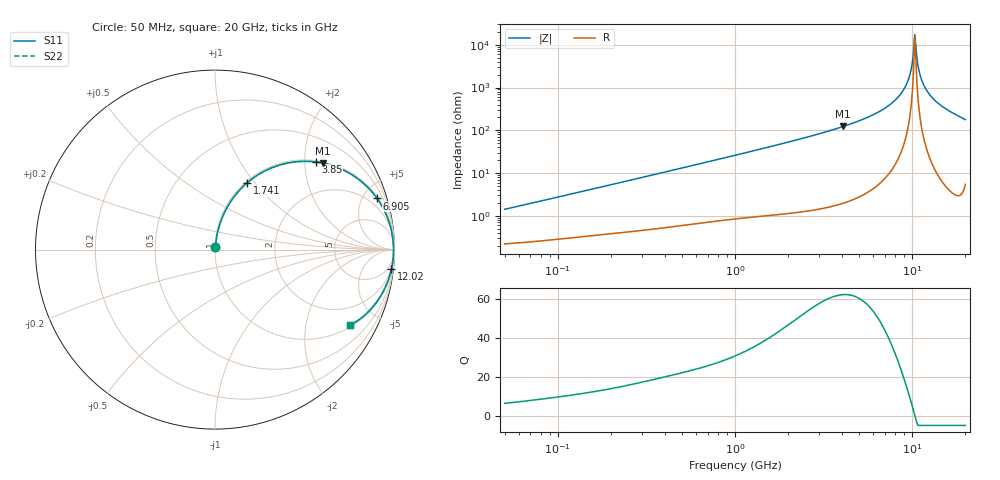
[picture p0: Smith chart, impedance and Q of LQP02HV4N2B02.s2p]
!Murata Part Number: LQP02HV4N2B02
!These Parameters are Measured in Series Mode Connection
!  o--[Z]--o
!Port1  Port2
!  o-------o
!Freq. Start=50[MHz] Stop=20[GHz], 401[Steps]
# Hz S RI R 50
!Freq.(Hz) S11(Real) S11(Imag) S21(Real) S21(Imag) S12(Real) S12(Imag) S22(Real) S22(Imag)
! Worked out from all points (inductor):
!   401 points, 50 MHz to 20 GHz, reference 50 ohm
!   read as one part in series: L = 4.42 nH near 51.52 MHz
!   highest Q = 62.3 at 4.088 GHz (marker M1), where L = 4.79 nH
!   self-resonance near 10.35 GHz
!   S11 on the Smith chart (normalised r, x): 50 MHz: 1.00, +0.03; 1.741 GHz: 1.02, +0.91; 3.85 GHz: 1.04, +2.27; 6.905 GHz: 1.14, +6.29; 12.02 GHz: 2, -18; 20 GHz: 1.11, -3.53
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5e7  0.0024 0.014  0.9976 -0.014  0.9976 -0.014  0.0024 0.014
1.364002e8  0.00457 0.0366  0.9954 -0.0366  0.9954 -0.0366  0.00457 0.0366
3.721004e8  0.0144 0.0959  0.9856 -0.0959  0.9856 -0.0959  0.0144 0.0959
1e9  0.07 0.2394  0.93 -0.2394  0.93 -0.2394  0.07 0.2394
1.740566e9  0.1787 0.3716  0.8213 -0.3716  0.8213 -0.3716  0.1787 0.3716
2.728004e9  0.3599 0.4711  0.6401 -0.4711  0.6401 -0.4711  0.3599 0.4711
3.850025e9  0.5619 0.4882  0.4381 -0.4882  0.4381 -0.4882  0.5619 0.4882
4.087748e9  0.6004 0.4819  0.3996 -0.4819  0.3996 -0.4819  0.6004 0.4819
5.515528e9  0.788 0.4001  0.212 -0.4001  0.212 -0.4001  0.788 0.4001
6.905011e9  0.903 0.2852  0.097 -0.2852  0.097 -0.2852  0.903 0.2852
7.442007e9  0.9325 0.2384  0.0675 -0.2384  0.0675 -0.2384  0.9325 0.2384
8.389408e9  0.9687 0.1569  0.0313 -0.1569  0.0313 -0.1569  0.9687 0.1569
9.178299e9  0.9859 0.0918  0.0141 -0.0918  0.0141 -0.0918  0.9859 0.0918
9.745021e9  0.9924 0.0473  0.00765 -0.0473  0.00765 -0.0473  0.9924 0.0473
1.019291e10  0.9946 0.0136  0.00544 -0.0136  0.00544 -0.0136  0.9946 0.0136
1.034674e10  0.9948 0.00236  0.00522 -0.00236  0.00522 -0.00236  0.9948 0.00236
1.066139e10  0.9945 -0.0202  0.00555 0.0202  0.00555 0.0202  0.9945 -0.0202
1.098561e10  0.9931 -0.0427  0.0069 0.0427  0.0069 0.0427  0.9931 -0.0427
1.115139e10  0.992 -0.0539  0.00797 0.0539  0.00797 0.0539  0.992 -0.0539
1.201863e10  0.9829 -0.1096  0.0171 0.1096  0.0171 0.1096  0.9829 -0.1096
1.460232e10  0.9301 -0.2462  0.0699 0.2462  0.0699 0.2462  0.9301 -0.2462
2e10  0.7509 -0.4174  0.2491 0.4174  0.2491 0.4174  0.7509 -0.4174
